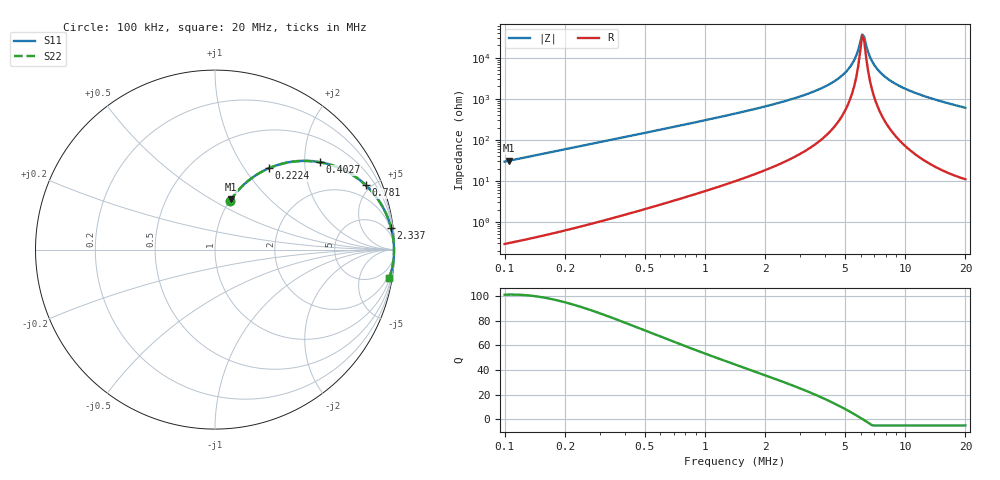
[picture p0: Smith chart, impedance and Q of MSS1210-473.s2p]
# MHz S MA R 50
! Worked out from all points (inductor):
!   233 points, 100 kHz to 20 MHz, reference 50 ohm
!   read as one part in series: L = 47 uH near 102.3 kHz
!   highest Q = 101 at 104.7 kHz (marker M1), where L = 47 uH
!   self-resonance near 6.099 MHz
!   S11 on the Smith chart (normalised r, x): 100 kHz: 1.01, +0.59; 222.4 kHz: 1.01, +1.31; 402.7 kHz: 1.03, +2.38; 781 kHz: 1.08, +4.65; 2.337 MHz: 2, +16; 20 MHz: 1, -12
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0.1  0.2825 73.0  0.9565 -16.4  0.9565 -16.4  0.2825 73.0
0.1046734  0.2945 72.3  0.9527 -17.1  0.9527 -17.1  0.2945 72.3
0.2224017  0.5455 56.3  0.8322 -33.1  0.8322 -33.1  0.5455 56.3
0.2436751  0.5803 53.9  0.808 -35.5  0.808 -35.5  0.5803 53.9
0.4027283  0.7602 39.8  0.64 -49.5  0.64 -49.5  0.7602 39.8
0.5937753  0.8636 29.4  0.4915 -59.7  0.4915 -59.7  0.8636 29.4
0.7809819  0.9131 23.1  0.3928 -65.9  0.3928 -65.9  0.9131 23.1
1.446882  0.9712 12.5  0.217 -76.2  0.217 -76.2  0.9712 12.5
2.337309  0.9884 7.1  0.1241 -81.1  0.1241 -81.1  0.9884 7.1
3.446086  0.9944 3.9  0.06799 -83.4  0.06799 -83.4  0.9944 3.9
4.430234  0.9964 2.1  0.03724 -83.4  0.03724 -83.4  0.9964 2.1
5.198215  0.9971 1.1  0.01898 -80.7  0.01898 -80.7  0.9971 1.1
5.695439  0.9973 0.5  0.008922 -72.5  0.008922 -72.5  0.9973 0.5
5.827005  0.9974 0.3  0.006517 -66.2  0.006517 -66.2  0.9974 0.3
6.099327  0.9974 0.1  0.002699 -19.1  0.002699 -19.1  0.9974 0.1
6.240223  0.9975 -0.1  0.003027 33.2  0.003027 33.2  0.9975 -0.1
6.531856  0.9975 -0.4  0.007205 69.4  0.007205 69.4  0.9975 -0.4
6.995058  0.9975 -0.8  0.01464 79.6  0.01464 79.6  0.9975 -0.8
7.491107  0.9974 -1.3  0.02231 82.6  0.02231 82.6  0.9974 -1.3
8.397251  0.997 -2.0  0.03542 84.2  0.03542 84.2  0.997 -2.0
11.56092  0.9949 -4.3  0.07511 84.0  0.07511 84.0  0.9949 -4.3
20  0.9838 -9.3  0.1623 79.6  0.1623 79.6  0.9838 -9.3
